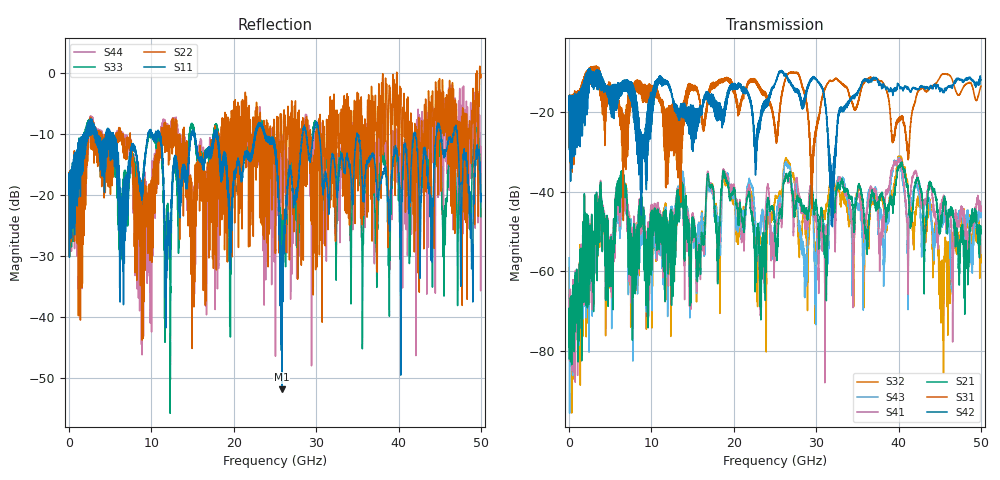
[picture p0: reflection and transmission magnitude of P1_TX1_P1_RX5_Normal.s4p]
!Keysight Technologies,N5225B,MY57041031,A.13.20.10
!Date: Friday, May 31, 2019 11:20:29
!Correction: S11(Full 4 Port(1,2,3,4))
!S12(Full 4 Port(1,2,3,4))
!S13(Full 4 Port(1,2,3,4))
!S14(Full 4 Port(1,2,3,4))
!S21(Full 4 Port(1,2,3,4))
!S22(Full 4 Port(1,2,3,4))
!S23(Full 4 Port(1,2,3,4))
!S24(Full 4 Port(1,2,3,4))
!S31(Full 4 Port(1,2,3,4))
!S32(Full 4 Port(1,2,3,4))
!S33(Full 4 Port(1,2,3,4))
!S34(Full 4 Port(1,2,3,4))
!S41(Full 4 Port(1,2,3,4))
!S42(Full 4 Port(1,2,3,4))
!S43(Full 4 Port(1,2,3,4))
!S44(Full 4 Port(1,2,3,4))
!S4P File: Measurements: <S11,S12,S13,S14>,
!<S21,S22,S23,S24>,
!<S31,S32,S33,S34>,
!<S41,S42,S43,S44>:
# Hz S  dB  R 50.0
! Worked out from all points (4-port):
!   5000 points, 10 MHz to 50 GHz, reference 50 ohm
!   strongest paths, dB at 10 MHz, 12.51 GHz, 25.01 GHz, 37.51 GHz, 50 GHz:
!     S42: -19.5, -15.7, -13.1, -12.4, -12.0
!     S31: -19.4, -29.3, -24.6, -11.8, -13.5
!     S21: -81.9, -48.3, -49.1, -42.8, -49.7
!     S41: -65.9, -46.1, -53.1, -46.6, -45.0
!     S43: -56.6, -45.6, -47.6, -46.9, -46.0
!     S32: -59.0, -46.9, -42.1, -43.2, -57.6
!   lowest |S11| = -51.9 dB at 25.83 GHz (marker M1), VSWR 1.01, Z = 50 + j0.254 ohm
!   |S11| at or under -10 dB: 18.01 GHz to 22.61 GHz (4.597 GHz wide, 22.6 % of centre); 30.38 GHz to 34.94 GHz (4.564 GHz wide, 14 % of centre); 34.97 GHz to 41.82 GHz (6.842 GHz wide, 17.8 % of centre)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
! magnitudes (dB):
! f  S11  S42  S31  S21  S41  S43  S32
! 10 MHz  -19.9  -19.5  -19.4  -81.9  -65.9  -56.6  -59.0
! 6.44 GHz  -21.9  -14.8  -28.4  -35.3  -37.5  -40.4  -37.4
! 23.21 GHz  -8.2  -21.2  -14.3  -56.5  -59.9  -50.2  -49.2
! 25.83 GHz  -51.9  -9.7  -16.0  -45.2  -47.6  -45.3  -40.2
! 31.94 GHz  -13.3  -36.3  -12.3  -41.4  -40.8  -39.1  -36.2
! 35.81 GHz  -20.0  -11.8  -12.7  -46.0  -50.5  -55.4  -66.7
! 50 GHz  -19.8  -12.0  -13.5  -49.7  -45.0  -46.0  -57.6
